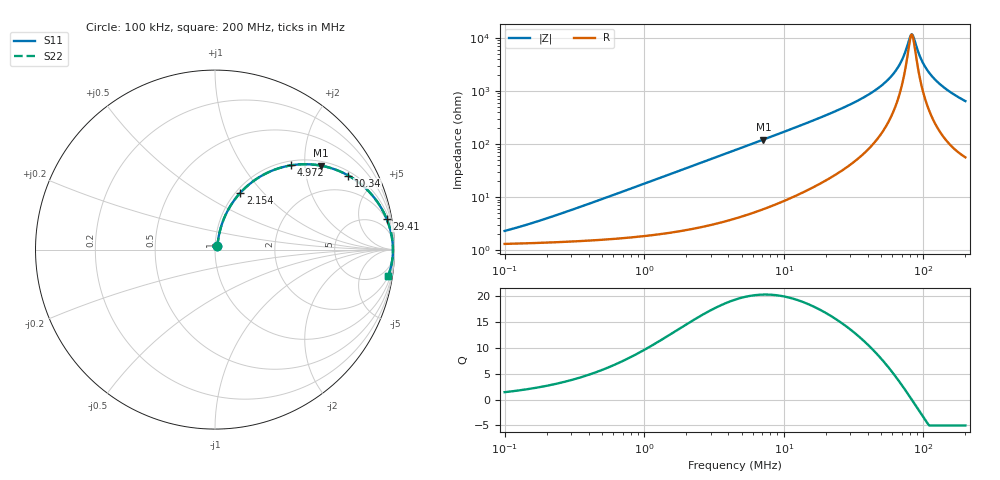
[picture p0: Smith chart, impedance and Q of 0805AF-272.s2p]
# MHz  S  MA  R  50
!Freq  MagS11  AngS11  MagS21  AngS21  MagS12  AngS12  MagS22  AngS22
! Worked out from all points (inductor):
!   801 points, 100 kHz to 200 MHz, reference 50 ohm
!   read as one part in series: L = 2.95 uH near 228.6 kHz
!   highest Q = 20.3 at 7.135 MHz (marker M1), where L = 2.7 uH
!   self-resonance near 82.08 MHz
!   S11 on the Smith chart (normalised r, x): 100 kHz: 1.03, +0.04; 2.154 MHz: 1.05, +0.75; 4.972 MHz: 1.09, +1.70; 10.34 MHz: 1.18, +3.50; 29.41 MHz: 2, +11; 200 MHz: 2, -13
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0.1  0.02295 54.2  0.9867 -1.1  0.9867 -1.1  0.02295 54.2
0.3573795  0.06645 73.4  0.9831 -3.7  0.9831 -3.7  0.06645 73.4
1.265119  0.2161 72.5  0.9574 -12.4  0.9574 -12.4  0.2161 72.5
2.15422  0.346 66.0  0.9156 -20.2  0.9156 -20.2  0.346 66.0
4.478507  0.595 50.6  0.7736 -36.5  0.7736 -36.5  0.595 50.6
4.972095  0.6328 47.9  0.7429 -39.2  0.7429 -39.2  0.6328 47.9
7.135051  0.7537 38.4  0.6212 -48.8  0.6212 -48.8  0.7537 38.4
10.33672  0.8503 29.0  0.4853 -58.1  0.4853 -58.1  0.8503 29.0
16.00527  0.9231 19.7  0.3371 -67.2  0.3371 -67.2  0.9231 19.7
29.40656  0.9711 10.2  0.1783 -75.6  0.1783 -75.6  0.9711 10.2
43.41955  0.9842 5.9  0.1026 -78.2  0.1026 -78.2  0.9842 5.9
56.65845  0.9889 3.3  0.05857 -77.4  0.05857 -77.4  0.9889 3.3
67.87245  0.9907 1.7  0.03101 -71.6  0.03101 -71.6  0.9907 1.7
72.5418  0.991 1.1  0.02144 -64.8  0.02144 -64.8  0.991 1.1
79.77498  0.9914 0.3  0.01005 -30.6  0.01005 -30.6  0.9914 0.3
82.86631  0.9914 -0.0  0.008609 3.9  0.008609 3.9  0.9914 -0.0
86.07744  0.9914 -0.4  0.01067 36.2  0.01067 36.2  0.9914 -0.4
92.87782  0.9913 -1.0  0.01988 63.5  0.01988 63.5  0.9913 -1.0
98.32841  0.9911 -1.5  0.02806 70.6  0.02806 70.6  0.9911 -1.5
113.3957  0.99 -2.8  0.04986 77.0  0.04986 77.0  0.99 -2.8
143.8111  0.9862 -5.1  0.08918 78.6  0.08918 78.6  0.9862 -5.1
200  0.9752 -8.7  0.1517 76.3  0.1517 76.3  0.9752 -8.7
